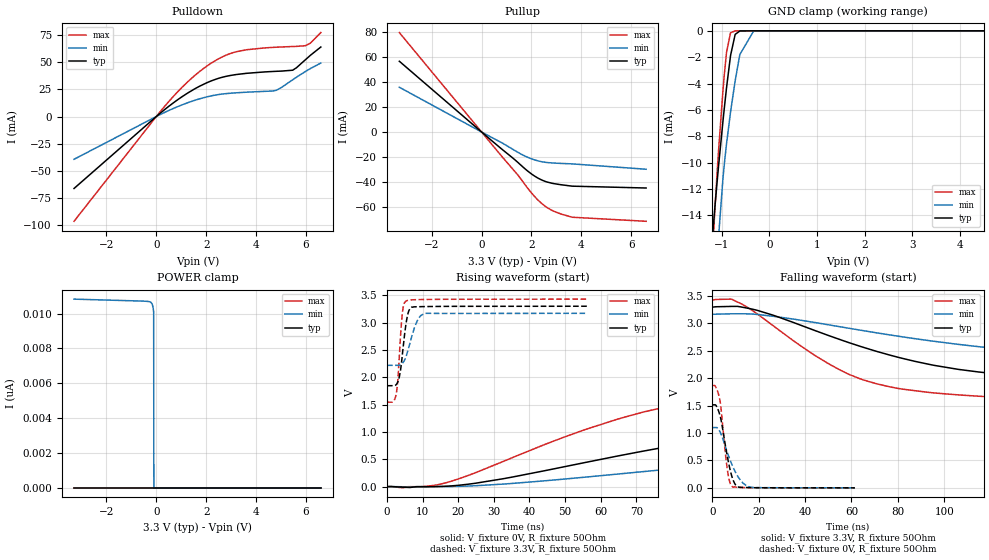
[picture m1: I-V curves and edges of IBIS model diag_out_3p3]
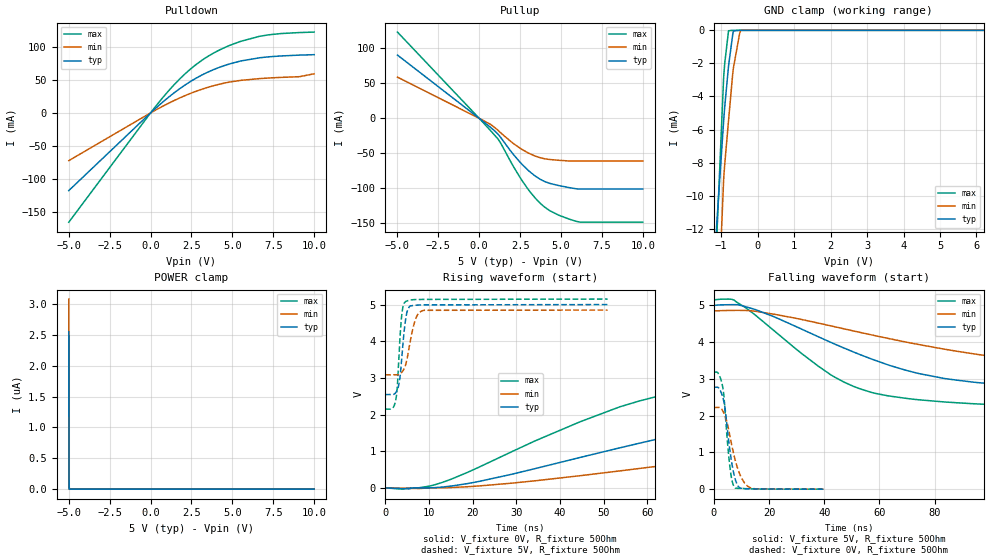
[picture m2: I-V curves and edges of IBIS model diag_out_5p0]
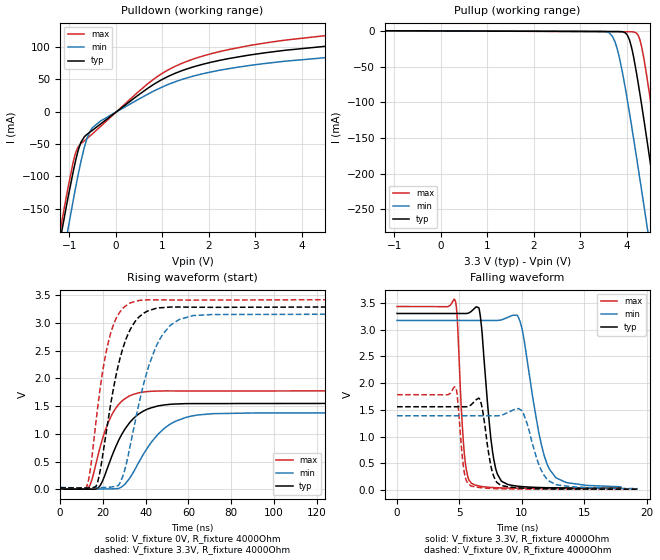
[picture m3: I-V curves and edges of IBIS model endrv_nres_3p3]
|Texas Instruments Incorporated
| Multi-Rail Power Supply for Microcontrollers in Safety-Critical Applications
| Marketing part#   Digital Voltage Range   Package-type   #pins
| TPS65381QDAPRQ1   3.0V-5.5V   HTSSOP   32
[IBIS Ver]   4.1
[File name]   tps65381-q1.ibs
[File Rev]   1.0
[Date]   12/9/2013
[Source]
| Texas Instruments Incorporated.
| Analog-eLab Design Center, HPA
| 12500 TI Blvd
| Dallas, TX -75243
[Notes]   Revision History:
| Rev 1.0: 12/9/2013
| - Initial version of the model
| - Model generated from simulations in TISPICE
| - Model matched to SPICE simulation
| - C_comp although listed in numerical order of value are
|   obtained from varying PVT conditions. For PVT conditions for
|   each specific value refer the buffer description under
|   respective [Model]. IBIS model user is responsible for using
|   appropriate C_comp to simulate for Signal Integrity.
|*  EXCEPTION:   *
|*  - For model endrv_nres_3p3 and endrv_nres_5p0,there will be a leakage*
|*   currents in the Pulldown IV-table because of the internal pullup   *
|*   resistor (RES_P1H) connected to the pad.   *
|*  - For model error, there will be a leakage current in the Powerclamp *
|*   IV-table because of the MN7 and MN6 devices connected between PAD  *
|*   and Ground are on.   *
|*  - For model sclk_sdi,there will be a leakage current in the   *
|*   PowerClamp IV-table because of the internal pulldown resistor   *
|*   (RES_P1H) connected to the pad   *
|*  - For model ncs_iovdd3p3 and ncs_iovdd5p0 there will be a leakage   *
|*   current in the GroundClamp IV-table because of the internal pullup *
|*   resistor (RES_P1H) connected to the pad   *
|*  - For model sel_vdd3_vdd5 tThere will be a leakage current in the   *
|*   GroundClamp IV-table because of the current source connected to   *
|*   the pad   *
[Disclaimer]
| This model is designed as an aid for customers of Texas Instruments.
| TI and its licensors and suppliers make no warranties, either expressed
| or implied, with respect to this  model, including the warranties of
| merchantability or fitness for a particular purpose. The model is
| provided solely on an "as is" basis. The entire risk as to its quality
| and performance is with the customer.
[Copyright]
(C) Copyright 2013 Texas Instruments Incorporated.All rights reserved.
|   TPS65381-Q1
[Component]   TPS65381-Q1
[Manufacturer]   TI
[Package]   |32 HTSSOP  -  DAP package
|   typ   min   max
R_pkg   0.005   NA   NA
L_pkg   0.20n   NA   NA
C_pkg   0.6p   NA   NA
[Pin]  signal_name   model_name   R_pin   L_pin   C_pin
1   VBAT_SAFING   nc   NA   NA   NA
2   VCP   nc   NA   NA   NA
3   CP1   nc   NA   NA   NA
4   CP2   nc   NA   NA   NA
5   PGND   gnd   NA   NA   NA
6   NRES   endrv_nres   NA   NA   NA
7   DIAG_OUT   diag_out   NA   NA   NA
8   NCS   ncs   NA   NA   NA
9   SDI   sclk_sdi   NA   NA   NA
10   SDO   sdo   NA   NA   NA
11   SCLK   sclk_sdi   NA   NA   NA
12   RSTEXT   nc   NA   NA   NA
13   ERROR/WDI   error   NA   NA   NA
14   CANWU   nc   NA   NA   NA
15   VSFB1   nc   NA   NA   NA
16   VSIN   nc   NA   NA   NA
17   VSOUT1   nc   NA   NA   NA
18   VTRACK1   nc   NA   NA   NA
19   GND   gnd   NA   NA   NA
20   VDD5   nc   NA   NA   NA
21   VDD3/5   nc   NA   NA   NA
22   VDDIO   power   NA   NA   NA
23   GND   gnd   NA   NA   NA
24   VDD1_SENSE   nc   NA   NA   NA
25   PGND   gnd   NA   NA   NA
26   VDD1_G   nc   NA   NA   NA
27   VDD6   nc   NA   NA   NA
28   SDN6   nc   NA   NA   NA
29   VBATP   power   NA   NA   NA
30   IGN   nc   NA   NA   NA
31   SEL_VDD3/5   sel_vdd3_vdd5   NA   NA   NA
32   ENDRV   endrv_nres   NA   NA   NA
|   Model Selectors
[Model Selector] endrv_nres
endrv_nres_3p3   3.3V  digital output
endrv_nres_5p0   5.0V  digital output
[Model Selector] diag_out
diag_out_3p3   3.3V  digital  tristate
diag_out_5p0   5.0V  digital  tristate
[Model Selector] ncs
ncs_iovdd3p3   3.3V  digital  input with VDDIO supply 3.3V
ncs_iovdd5p0   3.3V  digital  input with VDDIO supply 5.0V
[Model Selector] sdo
sdo_3p3   3.3V  digital I/O
sdo_5p0   5.0V  digital I/0
| Models and submodels in the file (11): diag_out_3p3 (3-state), diag_out_5p0 (3-state), endrv_nres_3p3 (Output), endrv_nres_5p0 (Output), error (Input), ncs_iovdd3p3 (Input), ncs_iovdd5p0 (Input), sclk_sdi (Input), sdo_3p3 (I/O), sdo_5p0 (I/O), sel_vdd3_vdd5 (Input)
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|   diag_out_3p3 Model
[Model]   diag_out_3p3
Model_type   3-state
Polarity   Non-Inverting
Vmeas = 1.65
Vref = 0
Cref = 2pF
Rref = 100
|   typ   min   max
|   (nom PVT)   (fast PVT)   (slow PVT)
C_comp   3.036e-12   2.744e-12   3.188e-12
| Where nom  PVT is Nominal Process, 3.3V, 27C
|   Fast PVT is Strong Process,  3.43V, -40C
|   Slow PVT is Weak Process,   3.17V, 150C
[Voltage Range]   3.3   3.17   3.43
|Junction Temperature
[Temperature Range]   27   150   -40
[Pullup Reference]   3.3   3.17   3.43
[Pulldown Reference]   0   0   0
[Power Clamp Reference]   3.3   3.17   3.43
[GND Clamp Reference]   0   0   0
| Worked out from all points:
|   slope of the pulldown table from 0 to 0.495 V, typ, clamps not added: 53.3 ohm
|   slope of the pullup table from 0 to 0.495 V, typ, clamps not added: 58.5 ohm
|   GND clamp passes 1 mA (typ) near -0.76 V on its own axis
|   falling waveform, V_fixture 3.3V, R_fixture 50Ohm: 20-80 % time 75.3ns typ, 113ns min, 45.8ns max; typ from 3.3 V to 1.85 V
|   rising waveform, V_fixture 0V, R_fixture 50Ohm: 20-80 % time 90.6ns typ, 142ns min, 52.2ns max; typ from 0 V to 1.51 V
|   rising waveform, V_fixture 3.3V, R_fixture 50Ohm: 20-80 % time 1.6ns typ, 2.65ns min, 1.12ns max; typ from 1.84 V to 3.3 V
|   falling waveform, V_fixture 0V, R_fixture 50Ohm: 20-80 % time 3.93ns typ, 6.21ns min, 2.73ns max; typ from 1.51 V to 0 V
[Pulldown]
|   Voltage   I(typ)   I(min)   I(max)
-3.3V     -66.14mA   -39.31mA   -96.32mA
257.4mV   4.95mA     2.92mA     7.254mA
1.025V    18.1mA     10.64mA    26.66mA
1.78V     28.34mA    16.55mA    42.14mA
2.49V     35.05mA    20.17mA    52.97mA
3.142V    38.36mA    21.69mA    59.13mA
3.633V    39.74mA    22.38mA    61.41mA
4.822V    41.57mA    24.17mA    63.72mA
5.468V    42.55mA    33.72mA    64.34mA
6.003V    52.64mA    41.67mA    65.27mA
6.174V    56.09mA    43.98mA    67.35mA
6.6V      63.9mA     49.17mA    77.17mA
[GND Clamp]
|   Voltage   I(typ)   I(min)   I(max)
-3.3V     -339.8mA   -348mA     -359.2mA
-1.262V   -18.68mA   -31.55mA   -21.26mA
-1.154V   -13.74mA   -21.56mA   -14.1mA
-1.068V   -10.27mA   -15.65mA   -9.09mA
-976.4mV  -6.876mA   -11.22mA   -4.559mA
-944.7mV  -5.775mA   -10.02mA   -3.215mA
-900.9mV  -4.322mA   -8.567mA   -1.64mA
-816.7mV  -1.876mA   -6.16mA    -148.2uA
-719.4mV  -270.1uA   -3.782mA   -3.491uA
-621.3mV  -13.48uA   -1.798mA   -107.1nA
-330mV    0A         -8.758uA   0A
6.6V      0A         0A         0A
[Pullup]
|   Voltage   I(typ)   I(min)   I(max)
-3.3V     56.84mA    35.95mA    79.89mA
855.9mV   -14.49mA   -9.161mA   -20.63mA
1.44V     -24.15mA   -16.15mA   -34.21mA
1.648V    -27.94mA   -18.41mA   -39.73mA
2.143V    -35.63mA   -22.51mA   -52.19mA
2.558V    -39.73mA   -24.35mA   -59.75mA
2.907V    -41.49mA   -24.95mA   -63.74mA
3.635V    -43.52mA   -25.62mA   -68.48mA
6.6V      -45mA      -29.92mA   -71.74mA
[POWER Clamp]
|   Voltage   I(typ)   I(min)   I(max)
-3.3V     0A         10.83nA    0A
-447mV    0A         10.71nA    0A
-257.6mV  0A         10.67nA    0A
-164.9mV  0A         10.53nA    0A
-126.8mV  0A         10.31nA    0A
-105.6mV  0A         10.08nA    0A
-98.3mV   0A         0A         0A
6.6V      0A         0A         0A
[Ramp]
R_load = 50
|   typ   min   max
dV/dt_r   0.908852/9.04547e-08   0.659401/1.41652e-07   1.1208/5.21138e-08
dV/dt_f   0.872618/7.50915e-08   0.570842/1.1314e-07   1.13161/4.55703e-08
[Falling Waveform]
V_fixture = 3.3V
V_fixture_min = 3.17V
V_fixture_max = 3.43V
R_fixture = 50Ohm
|   Time   V(typ)   V(min)   V(max)
0s        3.3V       3.17V      3.43V
8.25ns    3.312V     3.177V     3.445V
12.98ns   3.297V     3.177V     3.349V
44.45ns   2.868V     3.016V     2.41V
63.57ns   2.585V     2.88V      1.993V
81.9ns    2.364V     2.757V     1.803V
114.6ns   2.116V     2.578V     1.673V
184.9ns   1.939V     2.362V     1.582V
274.4ns   1.876V     2.271V     1.553V
750ns     1.846V     2.219V     1.544V
[Rising Waveform]
V_fixture = 0V
V_fixture_min = 0V
V_fixture_max = 0V
R_fixture = 50Ohm
|   Time   V(typ)   V(min)   V(max)
0s        408.8pV    189.7nV    311.5pV
11ns      -1.423mV   -7.484mV   3.488mV
17.35ns   9.128mV    1.327mV    84.31mV
55.55ns   439.6mV    172.2mV    1.041V
76.75ns   706.2mV    303.9mV    1.435V
94.87ns   902mV      413.4mV    1.609V
126.5ns   1.16V      584.1mV    1.725V
182.3ns   1.36V      814.5mV    1.808V
286.9ns   1.468V     1.005V     1.854V
750ns     1.515V     1.099V     1.868V
[Rising Waveform]
V_fixture = 3.3V
V_fixture_min = 3.17V
V_fixture_max = 3.43V
R_fixture = 50Ohm
|   Time   V(typ)   V(min)   V(max)
0s        1.845V     2.218V     1.544V
1.775ns   1.845V     2.219V     1.555V
2.625ns   1.868V     2.218V     1.709V
3.075ns   1.921V     2.218V     1.975V
4.275ns   2.389V     2.253V     3.147V
5.3ns     2.961V     2.371V     3.394V
6.6ns     3.267V     2.661V     3.415V
8.475ns   3.29V      3.03V      3.42V
10.38ns   3.293V     3.16V      3.423V
56.13ns   3.299V     3.169V     3.429V
[Falling Waveform]
V_fixture = 0V
V_fixture_min = 0V
V_fixture_max = 0V
R_fixture = 50Ohm
|   Time   V(typ)   V(min)   V(max)
0s        1.515V     1.101V     1.868V
1.425ns   1.512V     1.101V     1.847V
3.175ns   1.343V     1.034V     1.624V
3.775ns   1.241V     980.3mV    1.45V
6.675ns   531.4mV    623.8mV    284.5mV
7.75ns    318.5mV    500.6mV    79.39mV
8.9ns     152mV      383.4mV    14.26mV
11.4ns    12.36mV    183mV      10.05mV
16.2ns    4.388mV    14.75mV    3.357mV
61.42ns   272.6uV    334.1uV    219.5uV
|   diag_out_5p0 Model
[Model]   diag_out_5p0
Model_type   3-state
Polarity   Non-Inverting
Vmeas = 2.5
Vref = 0
Cref = 2pF
Rref = 100
|   typ   min   max
|   (nom PVT)   (fast PVT)   (slow PVT)
C_comp   3.078e-12   2.708e-12   3.211e-12
| Where nom  PVT is Nominal Process, 5V, 27C
|   Fast PVT is Strong Process,  5.15V, -40C
|   Slow PVT is Weak Process,   4.85V, 150C
[Voltage Range]   5   4.85   5.15
|Junction Temperature
[Temperature Range]   27   150   -40
[Pullup Reference]   5   4.85   5.15
[Pulldown Reference]   0   0   0
[Power Clamp Reference]   5   4.85   5.15
[GND Clamp Reference]   0   0   0
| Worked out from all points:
|   slope of the pulldown table from 0 to 0.75 V, typ, clamps not added: 45.4 ohm
|   slope of the pullup table from 0 to 0.75 V, typ, clamps not added: 53.4 ohm
|   GND clamp passes 1 mA (typ) near -0.73 V on its own axis
|   falling waveform, V_fixture 5V, R_fixture 50Ohm: 20-80 % time 54.5ns typ, 84.2ns min, 34.3ns max; typ from 5 V to 2.54 V
|   rising waveform, V_fixture 0V, R_fixture 50Ohm: 20-80 % time 68.6ns typ, 112ns min, 41.5ns max; typ from 0 V to 2.77 V
|   rising waveform, V_fixture 5V, R_fixture 50Ohm: 20-80 % time 1.17ns typ, 1.82ns min, 897ps max; typ from 2.54 V to 5 V
|   falling waveform, V_fixture 0V, R_fixture 50Ohm: 20-80 % time 2.86ns typ, 4.3ns min, 2.14ns max; typ from 2.77 V to 0.001 V
[Pulldown]
|   Voltage   I(typ)   I(min)   I(max)
-5V       -117.6mA   -72.31mA   -165.5mA
335mV     7.567mA    4.64mA     10.67mA
1.087V    23.46mA    14.42mA    33mA
1.788V    36.72mA    22.66mA    51.51mA
2.807V    52.91mA    32.95mA    73.68mA
3.347V    59.89mA    37.48mA    83.07mA
4.069V    67.66mA    42.56mA    93.44mA
5.506V    78.53mA    49.22mA    108.3mA
6.649V    83.41mA    51.88mA    115.9mA
7.24V     84.91mA    52.83mA    118.3mA
9.104V    87.47mA    54.8mA     121.6mA
10V       88.13mA    59.2mA     122.3mA
[GND Clamp]
|   Voltage   I(typ)   I(min)   I(max)
-5V       -708.4mA   -646.7mA   -791.2mA
-1.122V   -11.76mA   -19.13mA   -12.63mA
-1.12V    -11.67mA   -18.98mA   -12.52mA
-931.5mV  -5.47mA    -9.009mA   -2.852mA
-901.8mV  -4.632mA   -8.098mA   -1.991mA
-797.6mV  -2.157mA   -5.462mA   -24.62uA
-683.5mV  -263.3uA   -2.646mA   0A
-665mV    -38.1uA    -2.292mA   0A
-495mV    0A         -209.7uA   0A
-470.1mV  0A         -14.46uA   0A
-460.4mV  0A         0A         0A
10V       0A         0A         0A
[Pullup]
|   Voltage   I(typ)   I(min)   I(max)
-5V       90.43mA    58.91mA    123.3mA
102.2mV   -1.877mA   -1.218mA   -2.559mA
701mV     -13.07mA   -8.757mA   -17.81mA
1.149V    -22.56mA   -17.15mA   -29.56mA
1.35V     -28.57mA   -21.48mA   -37.04mA
2.05V     -50.49mA   -35.23mA   -67.16mA
2.634V    -66.13mA   -44.68mA   -89.48mA
3.4V      -82.03mA   -53.69mA   -113.3mA
4.036V    -90.58mA   -57.87mA   -127.5mA
4.894V    -96.21mA   -59.97mA   -138.7mA
6.206V    -101mA     -60.94mA   -148.4mA
10V       -101mA     -60.94mA   -148.4mA
[POWER Clamp]
|   Voltage   I(typ)   I(min)   I(max)
-5V       2.552uA    3.081uA    2.482uA
-4.995V   1.517uA    1.92uA     1.586uA
-4.995V   1.466uA    1.875uA    1.53uA
-4.99V    824.6nA    1.159uA    911.5nA
-4.985V   417.2nA    669.1nA    507.8nA
-4.985V   349.8nA    599.8nA    430.5nA
-4.98V    75.48nA    264.6nA    168.3nA
-4.979V   70.95nA    233.5nA    133.7nA
-4.976V   43.4nA     44.23nA    86.31nA
-4.969V   0A         13.91nA    0A
-4.966V   0A         0A         0A
10V       0A         0A         0A
[Ramp]
R_load = 50
|   typ   min   max
dV/dt_r   1.6633/6.85404e-08   1.3326/1.1178e-07   1.91001/4.14141e-08
dV/dt_f   1.47284/5.41618e-08   1.05937/8.38137e-08   1.8007/3.41907e-08
[Falling Waveform]
V_fixture = 5V
V_fixture_min = 4.85V
V_fixture_max = 5.15V
R_fixture = 50Ohm
|   Time   V(typ)   V(min)   V(max)
0s        5V         4.85V      5.15V
7.35ns    5.018V     4.862V     5.141V
15.13ns   4.882V     4.837V     4.728V
37.73ns   4.149V     4.519V     3.352V
50.78ns   3.725V     4.3V       2.791V
72.43ns   3.179V     3.96V      2.445V
93.87ns   2.912V     3.683V     2.324V
143.4ns   2.698V     3.341V     2.215V
231.7ns   2.59V      3.173V     2.164V
750ns     2.545V     3.084V     2.149V
[Rising Waveform]
V_fixture = 0V
V_fixture_min = 0V
V_fixture_max = 0V
R_fixture = 50Ohm
|   Time   V(typ)   V(min)   V(max)
0s        465.8pV    146.2nV    367.7pV
7.9ns     -1.859mV   -16.11mV   5.806mV
12.92ns   20.88mV    2.783mV    143.2mV
44.47ns   825.4mV    330.3mV    1.795V
62.58ns   1.338V     594.3mV    2.504V
80.4ns    1.792V     859.5mV    2.799V
106.8ns   2.251V     1.221V     2.967V
167.1ns   2.571V     1.794V     3.106V
253.3ns   2.701V     2.055V     3.161V
750ns     2.772V     2.221V     3.183V
[Rising Waveform]
V_fixture = 5V
V_fixture_min = 4.85V
V_fixture_max = 5.15V
R_fixture = 50Ohm
|   Time   V(typ)   V(min)   V(max)
0s        2.545V     3.084V     2.149V
2.45ns    2.602V     3.084V     2.414V
2.8ns     2.683V     3.086V     2.811V
3.275ns   2.916V     3.103V     3.848V
3.775ns   3.511V     3.149V     4.696V
4.675ns   4.593V     3.36V      5.082V
5.525ns   4.938V     3.858V     5.116V
6.825ns   4.98V      4.559V     5.135V
8.425ns   4.989V     4.829V     5.139V
50.93ns   4.999V     4.849V     5.149V
[Falling Waveform]
V_fixture = 0V
V_fixture_min = 0V
V_fixture_max = 0V
R_fixture = 50Ohm
|   Time   V(typ)   V(min)   V(max)
0s        2.773V     2.224V     3.183V
1.5ns     2.769V     2.224V     3.159V
3.225ns   2.501V     2.13V      2.772V
4.15ns    2.143V     1.971V     2.038V
5.725ns   1.106V     1.481V     663.1mV
6.55ns    688.8mV    1.174V     247mV
7.375ns   374.4mV    899.6mV    58.65mV
9.15ns    50.5mV     453.2mV    24.29mV
13.4ns    10.4mV     32.2mV     8.908mV
39.73ns   505.4uV    915.7uV    429.1uV
|   endrv_nres_3p3 Model
[Model]   endrv_nres_3p3
Model_type   Output
Polarity   Non-Inverting
Vmeas = 1.65
Vref = 1.65
Cref = 2pF
Rref = 50
|   typ   min   max
|   (nom PVT)   (fast PVT)   (slow PVT)
C_comp   1.872e-12   1.508e-12   2.070e-12
| Where nom  PVT is Nominal Process, 3.3V, 27C
|   Fast PVT is Strong Process,  3.43V, -40C
|   Slow PVT is Weak Process,   3.17V, 150C
[Voltage Range]   3.3   3.17   3.43
|Junction Temperature
[Temperature Range]   27   150   -40
[Pullup Reference]   3.3   3.17   3.43
[Pulldown Reference]   0   0   0
[Power Clamp Reference]   3.3   3.17   3.43
[GND Clamp Reference]   0   0   0
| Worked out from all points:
|   slope of the pulldown table from 0 to 0.495 V, typ, clamps not added: 18.3 ohm
|   slope of the pullup table from 0 to 0.495 V, typ, clamps not added: 4.48 kohm
|   falling waveform, V_fixture 3.3V, R_fixture 4000Ohm: 20-80 % time 766ps typ, 1.4ns min, 465ps max; typ from 3.3 V to 0.035 V
|   rising waveform, V_fixture 0V, R_fixture 4000Ohm: 20-80 % time 12ns typ, 15.1ns min, 9.26ns max; typ from 0.013 V to 1.55 V
|   rising waveform, V_fixture 3.3V, R_fixture 4000Ohm: 20-80 % time 10ns typ, 12.4ns min, 7.92ns max; typ from 0.028 V to 3.3 V
|   falling waveform, V_fixture 0V, R_fixture 4000Ohm: 20-80 % time 639ps typ, 1.15ns min, 417ps max; typ from 1.56 V to 0.017 V
[Pulldown]
|   Voltage   I(typ)   I(min)   I(max)
-3.3V     -1.141A    -1.169A    -1.144A
-1.195V   -196.5mA   -249.8mA   -181.9mA
-1.066V   -146mA     -195.9mA   -130.9mA
-1.023V   -129.9mA   -178.4mA   -114.5mA
-864.7mV  -74.88mA   -116.3mA   -63.15mA
-759mV    -48.36mA   -79.01mA   -49.81mA
-656.7mV  -37.16mA   -49.31mA   -43.56mA
-507.2mV  -28.72mA   -24.76mA   -34.3mA
697.4mV   36.75mA    27.49mA    43.85mA
1.417V    63.31mA    49.71mA    74.62mA
3.231V    91.22mA    74.72mA    106.4mA
6.6V      112.7mA    93.97mA    130.6mA
[Pullup]
|   Voltage   I(typ)   I(min)   I(max)
-3.3V     736.3uA    642.5uA    892.2uA
3.598V    -802.8uA   -1.869mA   -972.8uA
3.753V    -838.7uA   -15.51mA   -1.015mA
3.845V    -886uA     -37.12mA   -1.04mA
4.062V    -12.29mA   -114.4mA   -1.112mA
4.212V    -57.83mA   -175.5mA   -2.859mA
4.325V    -103.5mA   -223.4mA   -22.04mA
4.428V    -147.6mA   -267.5mA   -59.97mA
4.657V    -249.7mA   -366.8mA   -161.4mA
4.719V    -278mA     -394mA     -190.4mA
5.021V    -415mA     -525.9mA   -332.1mA
6.6V      -1.133A    -1.221A    -1.073A
[Ramp]
R_load = 4000
|   typ   min   max
dV/dt_r   0.925802/1.20186e-08   0.823646/1.51855e-08   1.0609/9.24766e-09
dV/dt_f   1.96174/7.63642e-10   1.87875/1.41764e-09   2.04112/4.65271e-10
[Falling Waveform]
V_fixture = 3.3V
V_fixture_min = 3.17V
V_fixture_max = 3.43V
R_fixture = 4000Ohm
|   Time   V(typ)   V(min)   V(max)
0s        3.3V       3.17V      3.43V
4.65ns    3.3V       3.17V      3.544V
5.4ns     3.299V     3.17V      654.5mV
5.95ns    3.34V      3.17V      126.2mV
6.6ns     3.355V     3.17V      73.91mV
7.525ns   939.4mV    3.17V      47.84mV
8.35ns    168.3mV    3.18V      39.41mV
9.85ns    66.84mV    3.153V     33.46mV
12.25ns   42.18mV    373.6mV    30.94mV
17.93ns   34.94mV    59.69mV    30.04mV
[Rising Waveform]
V_fixture = 0V
V_fixture_min = 0V
V_fixture_max = 0V
R_fixture = 4000Ohm
|   Time   V(typ)   V(min)   V(max)
0s        13.29mV    14.99mV    13.97mV
13.27ns   4.786mV    7.623mV    35.94mV
18.25ns   46.89mV    7.938mV    698.2mV
21.87ns   360.4mV    8.597mV    1.146V
25.75ns   747.1mV    12.86mV    1.449V
30.3ns    1.086V     94.37mV    1.634V
37.1ns    1.368V     510.1mV    1.743V
49.1ns    1.523V     1.112V     1.774V
64.73ns   1.546V     1.342V     1.772V
239.2ns   1.554V     1.384V     1.78V
[Rising Waveform]
V_fixture = 3.3V
V_fixture_min = 3.17V
V_fixture_max = 3.43V
R_fixture = 4000Ohm
|   Time   V(typ)   V(min)   V(max)
0s        28.17mV    34.23mV    26.88mV
12.2ns    23.52mV    28.57mV    33.26mV
14.32ns   26.9mV     29.4mV     413.1mV
16.83ns   58.1mV     30.71mV    1.245V
23.6ns    1.528V     41.03mV    2.811V
27.98ns   2.358V     116.7mV    3.197V
32.98ns   2.895V     831.8mV    3.361V
44.6ns    3.258V     2.552V     3.415V
55.68ns   3.285V     3.061V     3.411V
245.6ns   3.298V     3.166V     3.429V
[Falling Waveform]
V_fixture = 0V
V_fixture_min = 0V
V_fixture_max = 0V
R_fixture = 4000Ohm
|   Time   V(typ)   V(min)   V(max)
0s        1.556V     1.388V     1.782V
4.7ns     1.556V     1.388V     1.918V
5.35ns    1.556V     1.388V     382.6mV
6ns       1.608V     1.388V     70.31mV
6.675ns   1.665V     1.388V     44.59mV
7.55ns    410.9mV    1.387V     28.94mV
8.325ns   86.21mV    1.396V     23.2mV
9.975ns   36.46mV    1.486V     18.29mV
12.23ns   22.03mV    160.3mV    16.45mV
19.27ns   16.52mV    25.66mV    15.64mV
